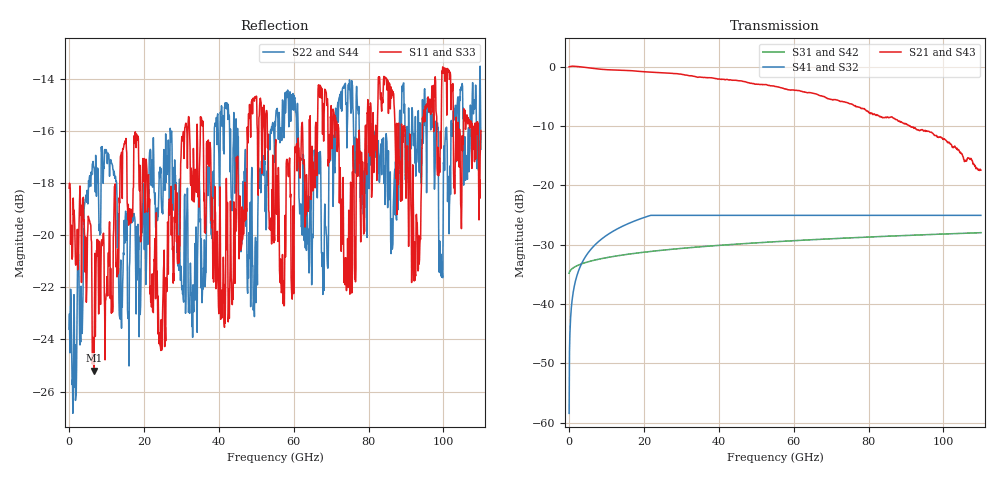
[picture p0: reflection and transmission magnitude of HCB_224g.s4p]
! Created with skrf 1.10.0 (http://scikit-rf.org).
# GHz S RI R 50.0
!freq ReS11 ImS11 ReS12 ImS12 ReS13 ImS13
! ReS14 ImS14
! ReS21 ImS21 ReS22 ImS22 ReS23 ImS23
! ReS24 ImS24
! ReS31 ImS31 ReS32 ImS32 ReS33 ImS33
! ReS34 ImS34
! ReS41 ImS41 ReS42 ImS42 ReS43 ImS43
! ReS44 ImS44
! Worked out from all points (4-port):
!   1101 points, 10 MHz to 110 GHz, reference 50 ohm
!   strongest paths, dB at 10 MHz, 27.51 GHz, 55.01 GHz, 82.5 GHz, 110 GHz:
!     S21: 0.0, -1.1, -3.3, -8.2, -17.4
!     S43: 0.0, -1.2, -3.3, -8.1, -17.3
!     S41: -58.4, -25.0, -25.0, -25.0, -25.0
!     S32: -58.4, -25.0, -25.0, -25.0, -25.0
!     S31: -34.8, -30.8, -29.5, -28.6, -28.0
!     S42: -34.8, -30.8, -29.5, -28.6, -28.0
!   lowest |S11| = -25.2 dB at 6.609 GHz (marker M1), VSWR 1.12, Z = 45 + j1.45 ohm
!   |S11| at or under -10 dB: start of sweep to end of sweep
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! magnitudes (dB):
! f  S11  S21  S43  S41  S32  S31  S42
! 10 MHz  -18.2  0.0  0.0  -58.4  -58.4  -34.8  -34.8
! 1.41 GHz  -19.2  0.1  0.0  -36.9  -36.9  -33.8  -33.8
! 6.609 GHz  -25.2  -0.3  -0.3  -30.2  -30.2  -32.6  -32.6
! 17.81 GHz  -16.5  -0.7  -0.7  -25.9  -25.9  -31.4  -31.4
! 24.41 GHz  -24.3  -1.0  -1.0  -25.0  -25.0  -30.9  -30.9
! 31.61 GHz  -17.4  -1.4  -1.4  -25.0  -25.0  -30.5  -30.5
! 110 GHz  -16.0  -17.4  -17.3  -25.0  -25.0  -28.0  -28.0
